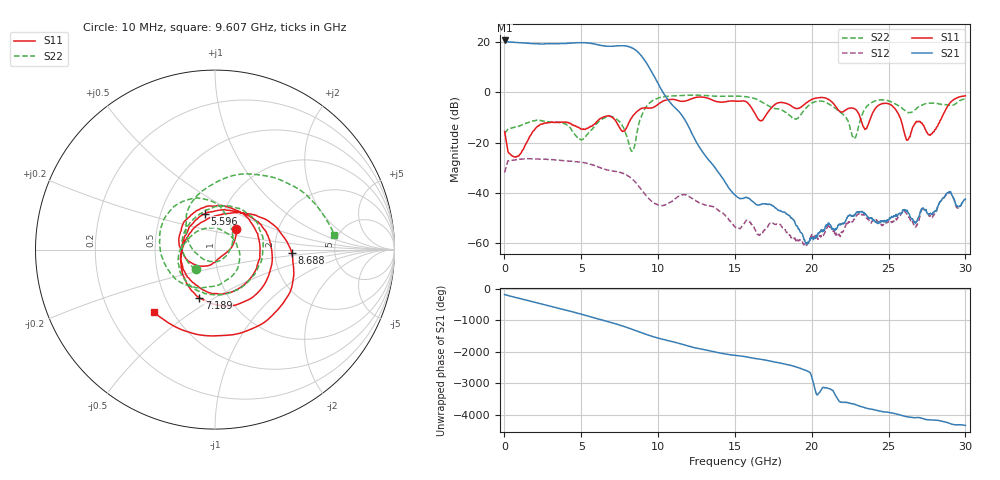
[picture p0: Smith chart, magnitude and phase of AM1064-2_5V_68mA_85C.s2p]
!Agilent	"Technologies,E8364B,MY43040894,A.07.50.67"
!Agilent	E8364B:	A.07.50.67
!Date:	"Wednesday,"	May	"01,"	2019	9:27:26
!Correction:	S11(Full	2	"Port(1,2))"
!S21(Full	2	"Port(1,2))"
!S12(Full	2	"Port(1,2))"
!S22(Full	2	"Port(1,2))"
!S2P	File:	Measurements:	"S11,"	"S21,"	"S12,"	S22:
#	Hz	S	dB	R	50
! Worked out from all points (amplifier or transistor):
!   1601 points, 10 MHz to 30 GHz, reference 50 ohm
!   highest |S21| = 20.5 dB at 10 MHz (marker M1)
!   |S21| within 3 dB of that: start of sweep to 8.313 GHz
!   unconditionally stable (mu >= 1): start of sweep to end of sweep
!   at 4.996 GHz: K = 1.44, MAG = 19.8 dB, |S12| = -27.8 dB
!   at 15.01 GHz: K = 4433.32, MAG = -33.1 dB, |S12| = -53.5 dB
!   at 30 GHz: K = 1266.55, MAG = -33.6 dB, |S12| = -43.2 dB
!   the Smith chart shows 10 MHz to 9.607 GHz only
!   S11 on the Smith chart (normalised r, x): 10 MHz: 1.23, +0.29; 5.596 GHz: 0.83, +0.34; 7.189 GHz: 0.73, -0.43; 8.688 GHz: 2.49, -0.13; 9.607 GHz: 0.40, -0.37
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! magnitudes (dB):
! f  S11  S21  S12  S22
! 10 MHz  -15.6  20.5  -31.9  -16.3
! 741 MHz  -25.8  19.7  -26.9  -13.8
! 2.428 GHz  -12.7  19.1  -26.6  -11.4
! 5.015 GHz  -14.7  19.6  -27.8  -19.0
! 5.596 GHz  -13.7  19.4  -28.6  -15.3
! 7.189 GHz  -11.0  18.3  -31.4  -10.2
! 8.295 GHz  -10.0  17.6  -34.4  -23.4
! 8.688 GHz  -7.4  15.9  -36.9  -14.2
! 9.607 GHz  -6.2  7.9  -43.4  -3.5
! 10.02 GHz  -4.8  3.1  -44.8  -2.3
! 11.8 GHz  -3.5  -11.6  -40.8  -1.3
! 15.01 GHz  -3.5  -40.8  -53.5  -1.6
! 16.69 GHz  -11.4  -44.5  -56.0  -3.7
! 18.92 GHz  -6.3  -52.1  -58.2  -10.7
! 20.01 GHz  -2.9  -57.8  -56.2  -4.3
! 22 GHz  -7.8  -52.1  -55.6  -8.6
! 22.76 GHz  -6.6  -49.0  -50.4  -18.5
! 23.5 GHz  -14.6  -48.3  -48.9  -6.3
! 25.01 GHz  -4.7  -50.6  -51.3  -3.5
! 26.25 GHz  -18.9  -47.5  -49.0  -8.1
! 27.81 GHz  -16.5  -48.4  -49.7  -4.3
! 30 GHz  -1.5  -42.4  -43.2  -2.7
